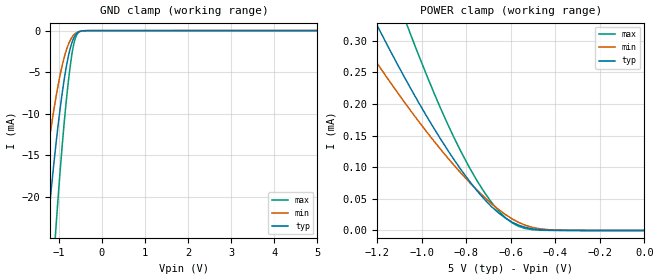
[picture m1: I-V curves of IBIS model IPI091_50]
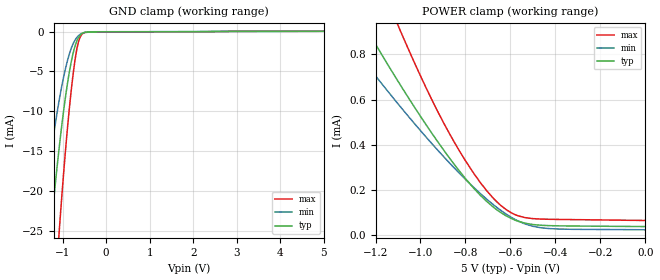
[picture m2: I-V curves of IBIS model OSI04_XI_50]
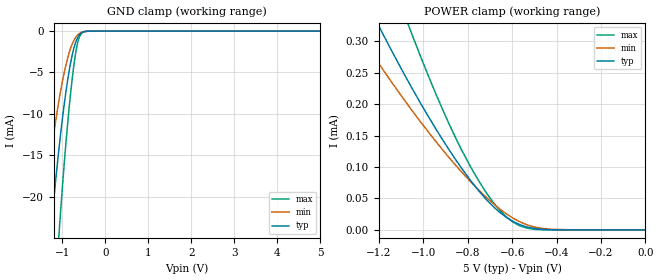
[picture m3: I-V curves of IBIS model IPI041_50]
| TEXAS INSTRUMENTS INCORPORATED
| Connectivity Solutions Group
| IBIS Model of TL16C2752FN_5V
| 2752FN_5V
| This file contains package information for the following:
|  FN 44-pin (PLCC) package as [Component] 2752FN_5V
| This device can be powered at the following Vccs:
|  5 volt Vcc
| This file provides unique models under the [Model Selector] for each Vcc.
| For operation at a specific Vcc, select the appropriate model after each
| [Model Selector] keyword.
[IBIS Ver]   3.2
[Comment char]  |_char
[File Name]   2752FN_5v.ibs
[File Rev]   1 | a
[Date]   August 8, 2006
[Source]   Data created from TI-SPICE simulations at TI-CONN.
[Notes]   The following is an IBIS list for the 2752FN_5V.
   Please contact s-ly@ti.com with questions and
   comments concerning CONN IBIS models.
[Disclaimer] Property of Texas Instruments Incorporated.  Unauthorized
   reproduction and/or distribution is strictly prohibited.
   This product is protected under copyright law.
   Created  2003, (C) Copyright  2003, Texas Instruments
   Incorporated, All Rights Reserved
   UNLESS THERE IS A SIGNED, WRITTEN AGREEMENT TO THE
   CONTRARY, TEXAS INSTRUMENTS (TI) IS PROVIDING THE IBIS
   MODELS  AND WITHOUT ANY WARRANTY, EXPRESSED OR
   IMPLIED.  TI assumes no liability for:
   1) the accuracy of the IBIS models provided to your
   company;
   2) the proper functioning of these IBIS Models in your
   design or for any resulting applications; or
   3) infringement of patents, copyrights or intellectual
   property rights resulting from your use of these IBIS
   models.
   TI provides IBIS Models as a service to our customers.
   You and your company shall not distribute, sell or give
   these models to anyone else without prior written
   permission from TI.
   TI reserves the right to make changes to our products or
   to discontinue any semiconductor product or service
   without notice, and advises our customers to obtain the
   latest version of relevant information to verify, before
   placing orders, that the information being relied on is
   current.
   Please be aware that your receipt and use of the IBIS
   information provided shall serve as acceptance of these
   terms and conditions.  If you do not accept these terms,
   you should return or destroy the IBIS models and any
   other accompanying information immediately.
| Component 2752_5V_PLCC 44-pin FN
[Component]   2752FN_5V
[Manufacturer]   Texas Instruments, Inc.
[Package]
|   typ   min   max
R_pkg   0.27365   0.25611   0.29119
L_pkg   3.46300n   3.21362n   3.71238n
C_pkg   0.17921p   0.17274p   0.18568p
[Pin]   signal_name   model_name   R_pin   L_pin   C_pin
1   TXRDYA   OPJ430   0.26610   3.35203n   0.17924p
2   D0   IPI04_OPJ43   0.25619   3.21362n   0.17274p
3   D1   IPI04_OPJ43   0.25703   3.22554n   0.17463p
4   D2   IPI04_OPJ43   0.26223   3.29838n   0.17902p
5   D3   IPI04_OPJ43   0.27188   3.43361n   0.18430p
6   D4   IPI04_OPJ43   0.28894   3.67285n   0.18405p
7   D5   IPI04_OPJ43   0.29092   3.70140n   0.18430p
8   D6   IPI04_OPJ43   0.27461   3.47357n   0.18401p
9   D7   IPI04_OPJ43   0.26580   3.35093n   0.17962p
10   A0   IPI041   0.26009   3.27164n   0.17623p
11   XTAL1   OSI04_XI   0.25816   3.24536n   0.17654p
12   GND   GND   0.26003   3.27223n   0.17871p
13   XTAL2   OSI04   0.25717   3.23295n   0.17470p
14   A1   IPI041   0.25762   3.23991n   0.17442p
15   A2   IPI041   0.26293   3.31463n   0.17955p
16   CHSEL   IPI041   0.27233   3.44671n   0.18401p
17   INTB   OPJ430   0.28853   3.67422n   0.18341p
18   CS   IPI041   0.28949   3.68860n   0.18516p
19   MFB   OPJ430   0.27189   3.44239n   0.18490p
20   IOW   IPI041   0.26222   3.30743n   0.17946p
21   RESET   IPI091   0.25694   3.23374n   0.17512p
22   GND   GND   0.25611   3.22234n   0.17417p
23   RTSB   OPJ430   0.25935   3.26764n   0.17611p
24   IOR   IPI041   0.25721   3.23771n   0.17415p
25   RXB   IPI041   0.25866   3.25783n   0.17500p
26   TXB   OPJ430   0.26418   3.33468n   0.18007p
27   DTRB   OPJ430   0.27430   3.47611n   0.18568p
28   CTSB   IPI041   0.29119   3.71238n   0.18515p
29   DSRB   IPI041   0.28780   3.66395n   0.18436p
30   CDB   IPI041   0.27039   3.41949n   0.18453p
31   RIB   IPI041   0.26088   3.28595n   0.17884p
32   TXRDYB   OPJ430   0.25629   3.22120n   0.17377p
33   VCC   POWER   0.25641   3.22223n   0.17297p
34   INTA   OPJ430   0.26011   3.27330n   0.17537p
35   MFA   OPJ430   0.25811   3.24463n   0.17410p
36   RTSA   OPJ430   0.25981   3.26771n   0.17557p
37   DTRA   OPJ430   0.26533   3.34432n   0.18028p
38   TXA   OPJ430   0.27534   3.48380n   0.18514p
39   RXA   IPI041   0.29078   3.69955n   0.18357p
40   CTSA   IPI041   0.28869   3.66932n   0.18288p
41   DSRA   IPI041   0.27269   3.44483n   0.18404p
42   CDA   IPI041   0.26282   3.30662n   0.17820p
43   RIA   IPI041   0.25821   3.24196n   0.17391p
44   VCC   POWER   0.25690   3.22349n   0.17422p
| Model IPI091
[Model Selector]   IPI091
IPI091_50   5 volt Vcc
| Model OSI04_XI
[Model Selector]   OSI04_XI
OSI04_XI_50   5 volt Vcc
| Model IPI041
[Model Selector]   IPI041
IPI041_50   5 volt Vcc
| Model IPI04_OPJ43
[Model Selector]   IPI04_OPJ43
IPI04_OPJ43_50   5 volt Vcc
| Model OPJ430
[Model Selector]   OPJ430
OPJ430_50   5 volt Vcc
| Model OSI04
[Model Selector]   OSI04
OSI04_50   5 volt Vcc
| Models and submodels in the file (6): IPI091_50 (Input), OSI04_XI_50 (Input), IPI041_50 (Input), IPI04_OPJ43_50 (I/O), OPJ430_50 (3-state), OSI04_50 (3-state)
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[Model]   IPI091_50
Model_type  Input
Vinl = 0
Vinh = 5
| variable   typ   min   max
C_comp   1.05pF   0.91pF   1.20pF
[Temperature Range]   40   125   -40
| Ambient temperature   25   110   -40
[Voltage range]   5   4.5   5.5
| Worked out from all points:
|   GND clamp passes 1 mA (typ) near -0.66 V on its own axis
|   POWER clamp passes 1 mA (typ) near -2.02 V on its own axis
[GND Clamp]
| IPI091_50
|   Voltage   I(typ)   I(min)   I(max)
-5V       -337.5mA   -249.9mA   -446.9mA
-1.485V   -37.43mA   -23.94mA   -59.12mA
-1.27V    -24.21mA   -14.96mA   -39.8mA
-1.085V   -14.44mA   -8.531mA   -24.93mA
-1.065V   -13.5mA    -7.923mA   -23.45mA
-920mV    -7.399mA   -4.126mA   -13.63mA
-845mV    -4.864mA   -2.644mA   -9.318mA
-775mV    -2.962mA   -1.595mA   -5.878mA
-665mV    -1.007mA   -578.3uA   -1.875mA
-570mV    -262.1uA   -185.2uA   -368.6uA
-400mV    -8.531uA   -12.92uA   -6.748uA
5V        489.4pA    4.684uA    103.1pA
[POWER Clamp]
| IPI091_50
|   Voltage   I(typ)   I(min)   I(max)
-5V       7.166mA    6.06mA     10.13mA
-1.305V   398.7uA    319.9uA    565.1uA
-1.185V   313.6uA    256.4uA    440.3uA
-1.08V    243.8uA    203.9uA    337.8uA
-1.045V   221.6uA    187.1uA    305.3uA
-915mV    144.4uA    128.2uA    193uA
-785mV    77.58uA    75.9uA     99.02uA
-715mV    47.95uA    51.41uA    58.45uA
-625mV    19.85uA    25.4uA     20.38uA
-565mV    8.395uA    12.83uA    6.553uA
-465mV    1.046uA    2.445uA    370.2nA
-84.4fV   489.4pA    3.799nA    117.2pA
[Model]   OSI04_XI_50
Model_type  Input
Vinl = 0
Vinh = 5
| variable   typ   min   max
C_comp   1.87pF   1.18pF   2.42pF
[Temperature Range]   40   125   -40
| Ambient temperature   25   110   -40
[Voltage range]   5   4.5   5.5
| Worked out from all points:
|   GND clamp passes 1 mA (typ) near -0.66 V on its own axis
|   POWER clamp passes 1 mA (typ) near -1.29 V on its own axis
[GND Clamp]
| OSI04_XI_50
|   Voltage   I(typ)   I(min)   I(max)
-5V       -343.1mA   -253.2mA   -455.7mA
-1.525V   -41.07mA   -26.37mA   -64.46mA
-1.48V    -38.05mA   -24.29mA   -60.12mA
-1.265V   -24.63mA   -15.21mA   -40.45mA
-1.085V   -14.94mA   -8.861mA   -25.7mA
-1.065V   -13.97mA   -8.241mA   -24.18mA
-915mV    -7.534mA   -4.251mA   -13.83mA
-770mV    -3.03mA    -1.696mA   -5.942mA
-665mV    -1.111mA   -697uA     -2.029mA
-565mV    -298uA     -251.7uA   -421.3uA
-390mV    -48.3uA    -40.46uA   -75.23uA
5V        38.17uA    39.29uA    59.24uA
[POWER Clamp]
| OSI04_XI_50
|   Voltage   I(typ)   I(min)   I(max)
-5V       11.35mA    8.695mA    16.41mA
-1.365V   1.132mA    919.8uA    1.585mA
-1.25V    930.2uA    769uA      1.291mA
-1.215V   870.6uA    724.2uA    1.204mA
-1.115V   705.4uA    599.5uA    963.5uA
-1.085V   657.4uA    563.1uA    893.9uA
-945mV    444.6uA    400.2uA    590.1uA
-800mV    250.3uA    246.8uA    329.3uA
-705mV    148.8uA    158.9uA    196uA
-620mV    86.09uA    93.87uA    113.7uA
-465mV    43.98uA    32.94uA    71.4uA
-84.4fV   38.17uA    24.06uA    65.18uA
[Model]   IPI041_50
Model_type  Input
Vinl = 0
Vinh = 5
| variable   typ   min   max
C_comp   1.06pF   0.91pF   1.20pF
[Temperature Range]   40   125   -40
| Ambient temperature   25   110   -40
[Voltage range]   5   4.5   5.5
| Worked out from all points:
|   GND clamp passes 1 mA (typ) near -0.66 V on its own axis
|   POWER clamp passes 1 mA (typ) near -2.02 V on its own axis
[GND Clamp]
| IPI041_50
|   Voltage   I(typ)   I(min)   I(max)
-5V       -337.5mA   -249.9mA   -446.9mA
-1.485V   -37.43mA   -23.94mA   -59.12mA
-1.27V    -24.21mA   -14.96mA   -39.8mA
-1.085V   -14.44mA   -8.531mA   -24.93mA
-1.065V   -13.5mA    -7.923mA   -23.45mA
-920mV    -7.399mA   -4.126mA   -13.63mA
-845mV    -4.864mA   -2.644mA   -9.318mA
-775mV    -2.962mA   -1.595mA   -5.878mA
-665mV    -1.007mA   -578.3uA   -1.875mA
-570mV    -262.1uA   -185.2uA   -368.6uA
-400mV    -8.531uA   -12.92uA   -6.748uA
5V        489.4pA    4.684uA    103.1pA
[POWER Clamp]
| IPI041_50
|   Voltage   I(typ)   I(min)   I(max)
-5V       7.166mA    6.06mA     10.13mA
-1.305V   398.7uA    319.9uA    565.1uA
-1.185V   313.6uA    256.4uA    440.3uA
-1.08V    243.8uA    203.9uA    337.8uA
-1.045V   221.6uA    187.1uA    305.3uA
-915mV    144.4uA    128.2uA    193uA
-785mV    77.58uA    75.9uA     99.02uA
-715mV    47.95uA    51.41uA    58.45uA
-625mV    19.85uA    25.4uA     20.38uA
-565mV    8.395uA    12.83uA    6.553uA
-465mV    1.046uA    2.445uA    370.2nA
-84.4fV   489.4pA    3.799nA    117.2pA
